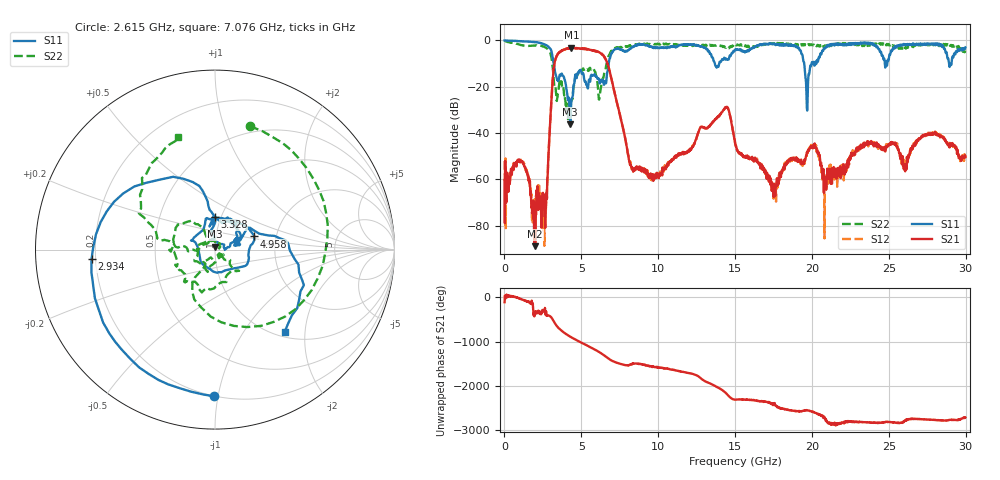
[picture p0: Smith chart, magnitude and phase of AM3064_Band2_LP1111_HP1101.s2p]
# Hz S DB R 50.0
!freq dBS11 angS11 dBS21 angS21 dBS12 angS12 dBS22 angS22
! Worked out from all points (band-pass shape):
!   1600 points, 10 MHz to 29.98 GHz, reference 50 ohm
!   highest |S21| = -3.23 dB at 4.359 GHz (marker M1); lowest = -88.8 dB at 1.997 GHz (marker M2)
!   |S21| within 3 dB of the highest: 3.442 GHz to 6.385 GHz (2.944 GHz wide, 59.9 % of centre)
!   lowest |S11| = -36.2 dB at 4.284 GHz (marker M3), VSWR 1.03, Z = 50 + j1.55 ohm
!   |S11| at or under -10 dB: 3.206 GHz to 6.782 GHz (3.576 GHz wide, 71.6 % of centre); 13.68 GHz to 13.97 GHz (284.7 MHz wide, 2.06 % of centre); 19.5 GHz to 19.98 GHz (479.8 MHz wide, 2.43 % of centre)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
!   |S22| runs from -34.0 to -0.1 dB; largest |S21 - S12| = 0.017
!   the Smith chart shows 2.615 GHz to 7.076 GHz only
!   S11 on the Smith chart (normalised r, x): 2.615 GHz: 0.20, -0.98; 2.934 GHz: 0.18, -0.04; 3.328 GHz: 0.93, +0.35; 4.958 GHz: 1.53, +0.24; 7.076 GHz: 1.08, -1.57
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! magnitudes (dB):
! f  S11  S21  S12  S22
! 10 MHz  0.0  -60.3  -52.0  -0.1
! 1.116 GHz  -0.4  -52.4  -52.3  -2.1
! 1.997 GHz  -0.7  -88.8  -68.9  -2.3
! 2.615 GHz  -1.7  -66.6  -72.4  -2.9
! 2.934 GHz  -3.2  -40.2  -40.2  -4.9
! 3.328 GHz  -14.7  -7.8  -7.8  -20.6
! 4.284 GHz  -36.2  -3.5  -3.3  -29.7
! 4.359 GHz  -25.9  -3.2  -3.2  -25.9
! 4.958 GHz  -12.8  -3.7  -3.5  -12.3
! 5.015 GHz  -14.0  -3.7  -3.5  -13.2
! 6.195 GHz  -18.6  -5.3  -5.3  -23.7
! 7.076 GHz  -4.4  -20.1  -19.9  -3.6
! 8.257 GHz  -3.2  -54.8  -55.4  -2.0
! 10 GHz  -3.3  -58.0  -57.9  -1.6
! 14.39 GHz  -8.1  -29.0  -28.8  -3.2
! 15 GHz  -4.1  -44.7  -44.2  -2.2
! 17.54 GHz  -1.7  -61.9  -64.9  -1.3
! 19.69 GHz  -30.3  -48.5  -48.8  -2.0
! 19.99 GHz  -9.6  -45.9  -46.0  -1.8
! 20.95 GHz  -3.0  -60.2  -58.1  -2.2
! 25 GHz  -8.2  -45.4  -44.7  -1.6
! 29.98 GHz  -3.0  -50.4  -50.7  -4.4
